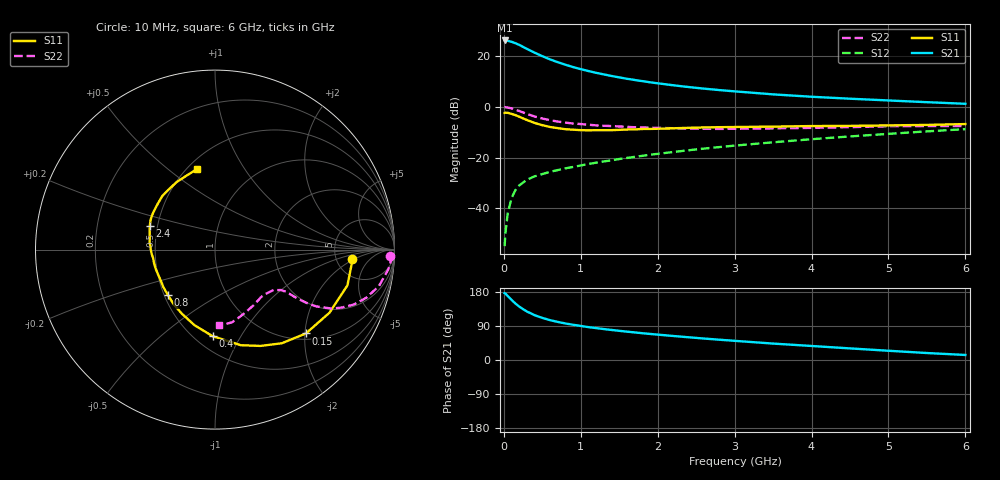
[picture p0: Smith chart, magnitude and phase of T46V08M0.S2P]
! Infineon Technologies  Discrete & RF Semiconductors
! BFR182T
! Si NPN RF Bipolar Junction Transistor in SC75
! VCE = 6 V  IC = 8 mA
! Common Emitter S-Parameters:  October  1999
# GHz  S  MA  R  50
!  f  S11  S21  S12  S22
! GHz  MAG  ANG  MAG  ANG  MAG  ANG  MAG  ANG
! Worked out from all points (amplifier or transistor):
!   36 points, 10 MHz to 6 GHz, reference 50 ohm
!   highest |S21| = 26.2 dB at 10 MHz (marker M1)
!   |S21| within 3 dB of that: start of sweep to 279.8 MHz
!   unconditionally stable (mu >= 1): 1.187 GHz to 3.956 GHz
!   at 250 MHz: K = 0.38, MSG = 26.7 dB, |S12| = -29.8 dB
!   at 1.4 GHz: K = 1.05, MAG = 15.3 dB, |S12| = -21.1 dB
!   at 6 GHz: K = 0.85, MSG = 5.0 dB, |S12| = -8.8 dB
!   lowest NFmin = 1.40 dB at 450 MHz
!   S11 on the Smith chart (normalised r, x): 10 MHz: 6.95, -1.81; 150 MHz: 1.14, -2.02; 400 MHz: 0.61, -0.77; 800 MHz: 0.52, -0.30; 2.4 GHz: 0.45, +0.14; 6 GHz: 0.56, +0.63
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0.01  0.7629 -4.1  20.4 176.5  0.0018 83.1  0.9764 -2.0
0.02  0.7675 -4.7  20.24 175.6  0.0032 95.6  0.9868 -2.6
0.05  0.7643 -15.1  20.12 168.8  0.0079 86.2  0.9715 -6.6
0.1  0.7283 -28.9  19.19 158.8  0.0159 78.4  0.9353 -12.6
0.15  0.6889 -42.7  18 149.1  0.0229 71.0  0.8839 -17.7
0.2  0.6409 -54.5  16.68 141.0  0.0283 67.8  0.8317 -21.6
0.25  0.5931 -64.8  15.23 134.1  0.0322 63.0  0.7758 -24.6
0.3  0.5517 -74.9  13.93 128.0  0.0368 61.4  0.7287 -26.8
0.4  0.4825 -91.6  11.73 118.2  0.0428 57.5  0.6467 -29.3
0.5  0.4364 -105.2  9.993 111.1  0.0474 57.4  0.5902 -30.2
0.6  0.4021 -117.3  8.641 105.2  0.0525 57.2  0.5474 -30.6
0.7  0.3816 -127.2  7.611 100.5  0.0569 57.9  0.5141 -30.7
0.8  0.364 -136.2  6.785 96.4  0.0615 58.1  0.4904 -30.7
1.1  0.3461 -157.4  5.09 86.7  0.075 60.5  0.445 -31.2
1.4  0.3478 -172.0  4.069 79.3  0.0885 61.9  0.419 -32.6
1.6  0.3585 179.8  3.588 74.8  0.0987 62.8  0.404 -33.7
2.2  0.3787 163.9  2.671 63.4  0.1292 64.1  0.3802 -39.4
2.4  0.3869 159.8  2.464 60.0  0.1398 64.1  0.3735 -41.7
3.5  0.4087 141.2  1.767 43.3  0.2007 62.3  0.3776 -55.5
4.5  0.4226 127.8  1.451 30.6  0.2619 58.5  0.3993 -69.7
5.5  0.4417 111.0  1.239 18.4  0.3293 53.5  0.4201 -82.1
6  0.4589 102.9  1.152 13.3  0.3649 50.1  0.4203 -87.1
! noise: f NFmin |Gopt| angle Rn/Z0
0.45  1.4  0.26  41  0.29
0.9  1.5  0.25  83  0.23
1.8  2  0.21  162  0.2
